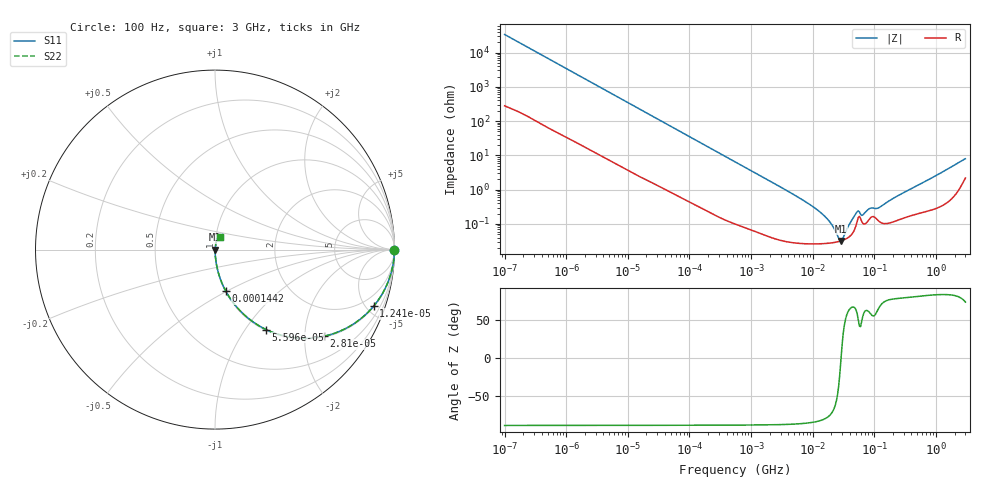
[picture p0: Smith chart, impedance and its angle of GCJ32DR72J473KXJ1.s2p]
!Murata Part Number: GCJ32DR72J473KXJ1
!These Parameters are Measured in Series Mode Connection
!Data Generated on Mar 13, 2026
!  o--ll--o
!Port1  Port2
!  o------o
!Operation Temp=25[degC], DC Bias Voltage=0[V]
!Freq. Start=100[Hz] Stop=3[GHz] 401[Steps]
# Hz S RI R 50
!Freq.(Hz) S11(Real) S11(Imag) S21(Real) S21(Imag) S12(Real) S12(Imag) S22(Real) S22(Imag)
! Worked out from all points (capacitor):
!   401 points, 100 Hz to 3 GHz, reference 50 ohm
!   read as one part in series: C = 47.1 nF near 109 Hz
!   lowest |Z| = 32 mohm at 28.73 MHz (marker M1)
!   series resonance near 28.82 MHz, so ESL is about 650 pH
!   S11 on the Smith chart (normalised r, x): 100 Hz: open; 12.4 kHz: 1.06, -5.61; 28.1 kHz: 1.03, -2.49; 55.95 kHz: 1.01, -1.26; 144.2 kHz: 1.01, -0.49; 3 GHz: 1.04, +0.15
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100  1 -0.00297  3.34e-05 0.00297  3.34e-05 0.00297  1 -0.00297
1788  0.9968 -0.0519  0.00322 0.0519  0.00322 0.0519  0.9968 -0.0519
5024  0.9779 -0.1419  0.0221 0.1419  0.0221 0.1419  0.9779 -0.1419
12405  0.8846 -0.3143  0.1154 0.3143  0.1154 0.3143  0.8846 -0.3143
28103  0.6065 -0.4829  0.3935 0.4829  0.3935 0.4829  0.6065 -0.4829
31977  0.5447 -0.4923  0.4553 0.4923  0.4553 0.4923  0.5447 -0.4923
55955  0.2853 -0.4457  0.7147 0.4457  0.7147 0.4457  0.2853 -0.4457
144239  0.0594 -0.2302  0.9406 0.2302  0.9406 0.2302  0.0594 -0.2302
547723  0.00522 -0.0648  0.9948 0.0648  0.9948 0.0648  0.00522 -0.0648
9794414  0.000272 -0.00329  0.9997 0.00329  0.9997 0.00329  0.000272 -0.00329
1.713898e7  0.000273 -0.00139  0.9997 0.00139  0.9997 0.00139  0.000273 -0.00139
2.12544e7  0.000284 -0.000796  0.9997 0.000796  0.9997 0.000796  0.000284 -0.000796
2.635803e7  0.000306 -0.000233  0.9997 0.000233  0.9997 0.000233  0.000306 -0.000233
2.872754e7  0.00032 -8.3e-06  0.9997 8.3e-06  0.9997 8.3e-06  0.00032 -8.3e-06
3.131008e7  0.000337 0.000221  0.9997 -0.000221  0.9997 -0.000221  0.000337 0.000221
4.0536e7  0.000446 0.000978  0.9996 -0.000978  0.9996 -0.000978  0.000446 0.000978
5.248048e7  0.00117 0.00194  0.9988 -0.00194  0.9988 -0.00194  0.00117 0.00194
6.508213e7  0.00104 0.00151  0.999 -0.00151  0.999 -0.00151  0.00104 0.00151
8.425944e7  0.00143 0.00244  0.9986 -0.00244  0.9986 -0.00244  0.00143 0.00244
1.138854e8  0.00128 0.00258  0.9987 -0.00258  0.9987 -0.00258  0.00128 0.00258
1.751444e8  0.00108 0.00463  0.9989 -0.00463  0.9989 -0.00463  0.00108 0.00463
3e9  0.0268 0.0729  0.9732 -0.0729  0.9732 -0.0729  0.0268 0.0729
